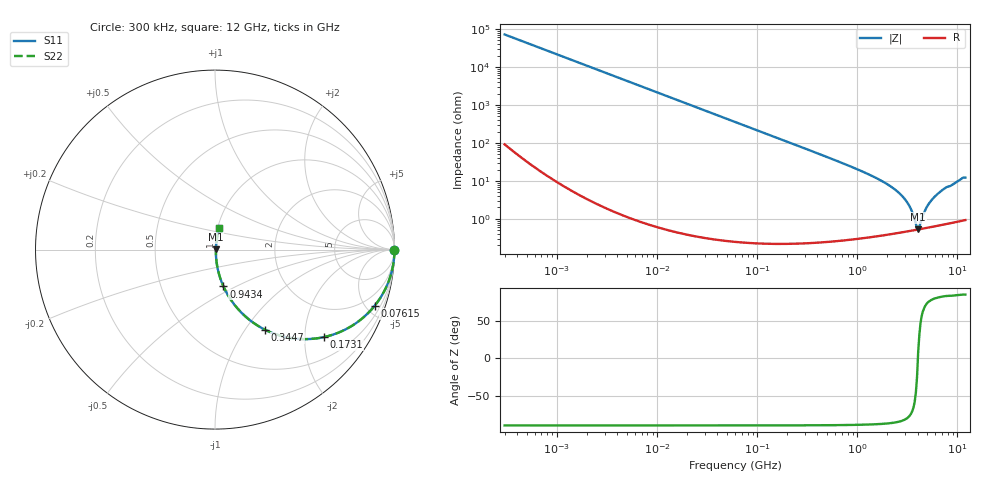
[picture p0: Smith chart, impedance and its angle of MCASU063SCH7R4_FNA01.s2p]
! MCASU063SCH7R4_FNA01  S-PARAMETER MODEL  ( General Type )
! Model Generated by TAIYO YUDEN Corporation (http://www.ty-top.com)
! Version 1.0
! TAIYO YUDEN Control No. 130801
! Copyright(c) 2013 TAIYO YUDEN CO.,LTD. All Rights Reserved.
! Product Description (link to TY-COMPAS)
! https://ds.yuden.co.jp/TYCOMPAS/or/detail?pn=MCASU063SCH7R4DFNA01&u=M
! Products Name : Multilayer Ceramic Capacitors
! Characteristics :
!  Capacitance : 7.4 pF , Rated Voltage : 50V , TCC : CH / C0H
!  Case Size : 0.6 x 0.3 / 0.024 x 0.012 [mm/inch] , Thickness : 0.3 / 0.012 [mm/inch]
!  (Conditions: Temperature = 25 degC , DC Bias Current/Voltage = 0A / 0V)
! External Node Assignments :
!  1  o---| |---o  2
! GND o---------o GND
! Frequency Range : 0.3MHz  -  12000MHz  [ 401 STEP ]
# MHz S RI R 50
! Freq[MHz].  S11 Real  S11 Imag  S21 Real  S21 Imag  S12 Real  S12 Imag  S22 Real  S22 Imag
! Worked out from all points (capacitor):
!   401 points, 300 kHz to 12 GHz, reference 50 ohm
!   read as one part in series: C = 7.37 pF near 316.3 kHz
!   lowest |Z| = 532 mohm at 4.05 GHz (marker M1)
!   series resonance near 4.026 GHz, so ESL is about 210 pH
!   S11 on the Smith chart (normalised r, x): 300 kHz: open; 76.15 MHz: 1.00, -5.67; 173.1 MHz: 1.00, -2.49; 344.7 MHz: 1.00, -1.24; 943.4 MHz: 1.01, -0.43; 12 GHz: 1.02, +0.24
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0.3  1 -0.00139  3.71e-06 0.00139  3.71e-06 0.00139  1 -0.00139
1.769972  0.9999 -0.0082  6.99e-05 0.0082  6.99e-05 0.0082  0.9999 -0.0082
10.44266  0.9977 -0.0483  0.00235 0.0483  0.00235 0.0483  0.9977 -0.0483
27.10171  0.9844 -0.1236  0.0156 0.1236  0.0156 0.1236  0.9844 -0.1236
60  0.9281 -0.258  0.0719 0.258  0.0719 0.258  0.9281 -0.258
76.15486  0.889 -0.3137  0.111 0.3137  0.111 0.3137  0.889 -0.3137
173.124  0.6075 -0.4874  0.3925 0.4874  0.3925 0.4874  0.6075 -0.4874
344.7396  0.2794 -0.4469  0.7206 0.4469  0.7206 0.4469  0.2794 -0.4469
353.9943  0.2688 -0.4414  0.7312 0.4414  0.7312 0.4414  0.2688 -0.4414
555.3718  0.1286 -0.3314  0.8714 0.3314  0.8714 0.3314  0.1286 -0.3314
943.3804  0.0472 -0.2055  0.9528 0.2055  0.9528 0.2055  0.0472 -0.2055
2088.533  0.00952 -0.0747  0.9905 0.0747  0.9905 0.0747  0.00952 -0.0747
2650.866  0.00642 -0.0458  0.9936 0.0458  0.9936 0.0458  0.00642 -0.0458
3107.553  0.00542 -0.028  0.9946 0.028  0.9946 0.028  0.00542 -0.028
3454.93  0.00514 -0.0166  0.9949 0.0166  0.9949 0.0166  0.00514 -0.0166
3841.137  0.00514 -0.00527  0.9949 0.00527  0.9949 0.00527  0.00514 -0.00527
4050.141  0.00524 0.000743  0.9948 -0.000743  0.9948 -0.000743  0.00524 0.000743
4270.516  0.00541 0.00572  0.9946 -0.00572  0.9946 -0.00572  0.00541 0.00572
5006.236  0.00626 0.0209  0.9937 -0.0209  0.9937 -0.0209  0.00626 0.0209
5868.704  0.00765 0.0366  0.9923 -0.0366  0.9923 -0.0366  0.00765 0.0366
7448.838  0.011 0.0622  0.989 -0.0622  0.989 -0.0622  0.011 0.0622
12000  0.0236 0.1183  0.9764 -0.1183  0.9764 -0.1183  0.0236 0.1183
